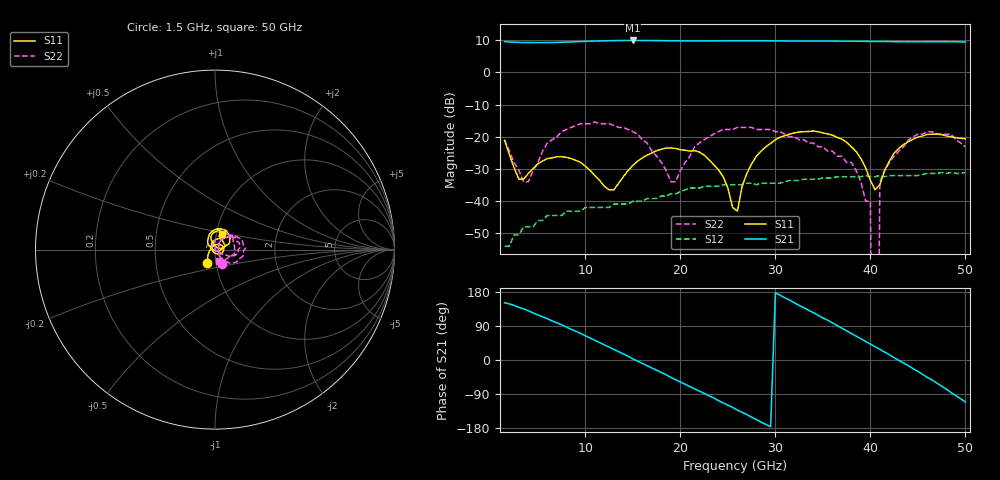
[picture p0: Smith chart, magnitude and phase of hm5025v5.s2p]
! HMMC-5025
! S-PARAMETERS  at  Vdd = 5V;  Idd = 75mA.  LAST UPDATED  02-07-97
#  GHZ  S  MA  R  50
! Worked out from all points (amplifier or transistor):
!   98 points, 1.5 GHz to 50 GHz, reference 50 ohm
!   highest |S21| = 9.9 dB at 15 GHz (marker M1)
!   |S21| within 3 dB of that: start of sweep to end of sweep
!   unconditionally stable (mu >= 1): start of sweep to end of sweep
!   at 9.5 GHz: K = 23.02, MAG = 9.7 dB, |S12| = -43.1 dB
!   at 26 GHz: K = 8.81, MAG = 9.9 dB, |S12| = -34.9 dB
!   at 50 GHz: K = 5.98, MAG = 9.5 dB, |S12| = -31.1 dB
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1.5  0.088 -119.0  3.02 151.0  0.002 -97.0  0.09 -65.0
4  0.027 81.0  2.92 130.0  0.004 -146.0  0.02 20.0
7.5  0.049 1.0  2.95 93.0  0.006 162.0  0.12 41.0
10  0.035 -44.0  3.04 64.0  0.008 132.0  0.16 14.0
13  0.015 -168.0  3.12 28.0  0.009 103.0  0.15 -18.0
15  0.036 121.0  3.14 3.0  0.01 86.0  0.12 -38.0
18  0.064 71.0  3.12 -33.0  0.012 61.0  0.04 -53.0
19.5  0.066 51.0  3.1 -52.0  0.013 47.0  0.02 27.0
22  0.058 21.0  3.09 -82.0  0.016 18.0  0.08 52.0
26  0.007 -164.0  3.1 -132.0  0.018 -28.0  0.14 16.0
27.5  0.038 147.0  3.1 -151.0  0.019 -46.0  0.14 4.0
30  0.09 111.0  3.09 177.0  0.019 -73.0  0.12 -13.0
34  0.123 61.0  3.07 125.0  0.022 -122.0  0.08 -26.0
37  0.092 27.0  3.06 84.0  0.024 -165.0  0.05 -32.0
40  0.021 22.0  3.03 42.0  0.024 157.0  0.01 -34.0
40.5  0.015 45.0  3.03 35.0  0.024 146.0  0 69.0
41  0.018 80.0  3.03 28.0  0.025 138.0  0.02 89.0
42  0.042 108.0  3.02 14.0  0.025 122.0  0.04 93.0
44  0.084 103.0  3.01 -15.0  0.025 97.0  0.09 70.0
45.5  0.103 84.0  3 -38.0  0.026 75.0  0.11 49.0
48  0.103 69.0  3.01 -77.0  0.027 32.0  0.11 -3.0
50  0.093 66.0  2.97 -111.0  0.028 -5.0  0.07 -70.0
